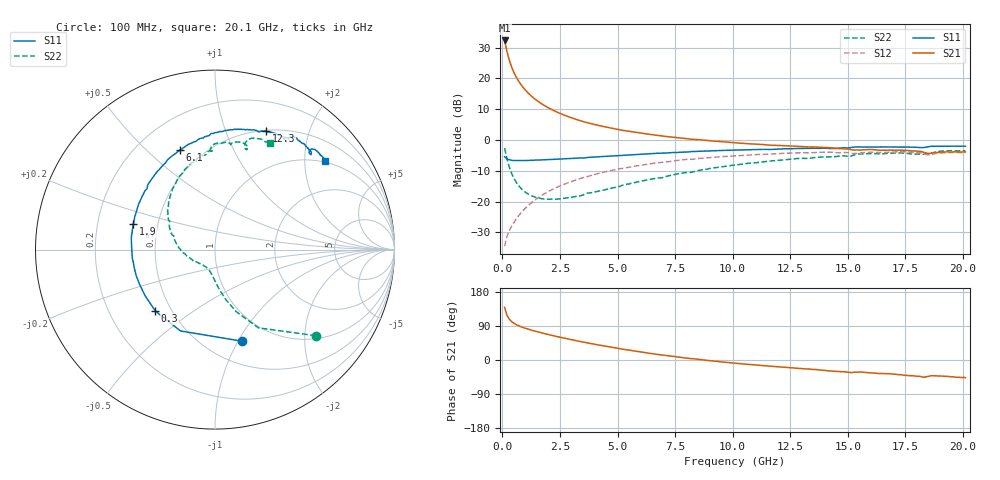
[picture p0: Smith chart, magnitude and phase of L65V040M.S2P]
!  Infineon Technologies AG
! BFR380L3 , PF131585-7, No.6, Th 09.10.01, soldered on pcb-board, measured with PP GSG850
!  Vce=5.0 V,  Ic=40.0 mA
! Common Emitter S-Parameters:  15. November 2001
#  GHz  S  MA  R  50
! f  S11  S21  S12  S22
! GHz  Mag  Ang  Mag  Ang  Mag  Ang  Mag  Ang
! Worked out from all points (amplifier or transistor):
!   201 points, 100 MHz to 20.1 GHz, reference 50 ohm
!   highest |S21| = 32.3 dB at 100 MHz (marker M1)
!   |S21| within 3 dB of that: start of sweep to 185.7 MHz
!   unconditionally stable (mu >= 1): 1.109 GHz to 4.315 GHz
!   at 3.4 GHz: K = 1.02, MAG = 8.5 dB, |S12| = -12.5 dB
!   at 10.1 GHz: K = 0.95, MSG = 2.1 dB, |S12| = -5.1 dB
!   at 20.1 GHz: K = 0.98, MSG = 0.1 dB, |S12| = -4.1 dB
!   S11 on the Smith chart (normalised r, x): 100 MHz: 0.73, -1.04; 300 MHz: 0.41, -0.36; 1.9 GHz: 0.36, +0.13; 6.1 GHz: 0.38, +0.64; 12.3 GHz: 0.51, +1.40; 20.1 GHz: 0.95, +2.52
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0.1  0.5324 -73.5  41.23 139.0  0.01882 61.8  0.7376 -40.5
0.2  0.4923 -113.0  27.56 118.4  0.02696 56.6  0.4989 -60.9
0.3  0.4772 -134.2  19.93 108.0  0.03334 57.4  0.3655 -71.1
0.4  0.4666 -146.8  15.45 101.6  0.03954 59.8  0.2879 -77.5
0.5  0.4626 -155.3  12.55 97.0  0.04528 61.9  0.239 -82.1
0.6  0.4624 -161.8  10.56 93.5  0.05175 63.6  0.206 -85.7
0.7  0.4613 -166.9  9.115 90.6  0.05808 64.8  0.1823 -88.9
0.8  0.4607 -170.8  8.017 88.0  0.06459 65.8  0.1649 -91.7
1  0.4631 -177.7  6.463 83.7  0.07779 67.0  0.1416 -96.8
1.2  0.4657 176.9  5.416 79.9  0.09122 67.4  0.1276 -101.6
1.5  0.4717 170.1  4.368 74.8  0.1114 67.2  0.1155 -108.4
1.9  0.4775 162.5  3.489 68.6  0.1385 65.9  0.1095 -117.3
2.6  0.4921 151.0  2.602 58.8  0.1852 62.6  0.112 -132.2
3.5  0.5087 138.2  1.99 47.3  0.2439 57.2  0.1271 -147.5
4.6  0.5432 125.0  1.59 34.9  0.3114 50.1  0.1604 -167.2
6.1  0.5888 109.4  1.278 20.2  0.3936 39.9  0.2173 171.5
6.8  0.607 102.7  1.175 14.0  0.429 34.8  0.2414 162.3
10.1  0.6843 78.3  0.8985 -8.3  0.5528 13.1  0.3918 129.3
12.3  0.7199 66.6  0.8037 -19.4  0.608 -0.6  0.4795 110.0
13.5  0.7315 60.8  0.7658 -24.8  0.623 -7.8  0.5131 101.2
16.8  0.7674 48.1  0.6841 -36.1  0.6315 -24.0  0.6078 79.6
20.1  0.7898 38.9  0.639 -46.5  0.6259 -37.9  0.669 63.0
